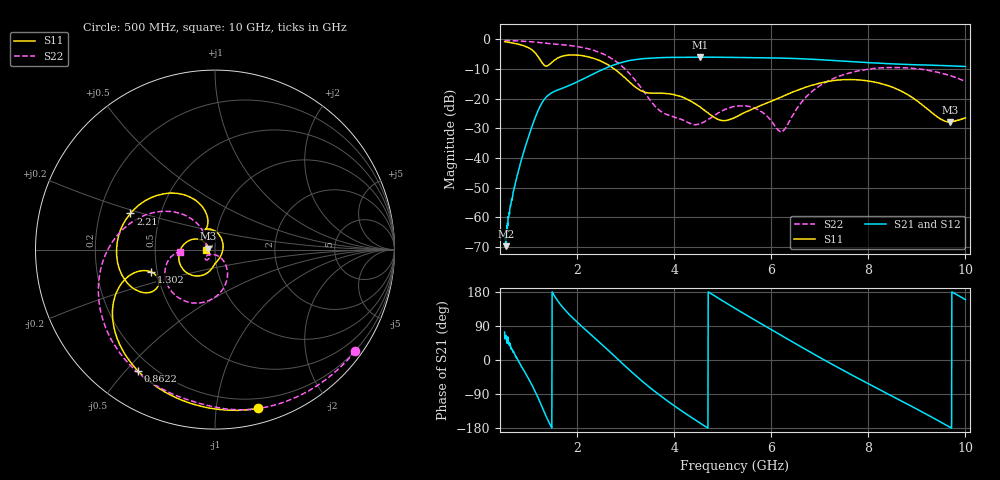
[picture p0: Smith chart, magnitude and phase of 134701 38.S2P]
!  2-Port S-parameters saved by WinCal
! VAR MeasName=S-Parameters (CALIBRATED_DATA) read from VNA (N5242A)
! VAR MeasDate=2013-7-3 16:37:20
! VAR NAME=134701 38
! VAR FILENAME=134701 38.S2P
! VAR DATE=2013-7-3 16:37:20
! VAR PHYS_PORTS=1,2
# Hz S MA R 50
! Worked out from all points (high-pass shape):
!   1601 points, 500 MHz to 10 GHz, reference 50 ohm
!   highest |S21| = -5.95 dB at 4.526 GHz (marker M1); lowest = -69.7 dB at 523.8 MHz (marker M2)
!   |S21| within 3 dB of the highest: 2.689 GHz to 9.74 GHz (7.051 GHz wide, 113 % of centre)
!   lowest |S11| = -27.8 dB at 9.679 GHz (marker M3), VSWR 1.08, Z = 46.1 + j0.538 ohm
!   |S11| at or under -10 dB: 2.768 GHz to end of sweep
!   |S22| runs from -31.1 to -0.3 dB; largest |S21 - S12| = 0.0022
!   S11 on the Smith chart (normalised r, x): 500 MHz: 0.12, -1.30; 862.2 MHz: 0.14, -0.54; 1.302 GHz: 0.46, -0.13; 2.21 GHz: 0.33, +0.18; 10 GHz: 0.91, -0.00
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5e8  0.9177 -74.7  0.0005114 73.8  0.0003456 81.2  0.9633 -35.9
5.2375e8  0.9114 -77.9  0.0003263 58.4  0.0005193 47.3  0.9615 -37.6
6.425e8  0.8793 -93.9  0.00202 27.8  0.001907 31.7  0.9547 -46.0
8.621875e8  0.8004 -122.5  0.01042 -19.9  0.0103 -20.5  0.9379 -61.6
1.075938e9  0.6564 -150.2  0.03632 -69.0  0.03631 -69.2  0.9131 -76.9
1.301562e9  0.3781 -160.9  0.09357 -132.9  0.09339 -133.0  0.8705 -92.4
1.598438e9  0.489 -152.0  0.1412 155.5  0.1408 155.2  0.8287 -111.9
2.085312e9  0.5356 167.2  0.2089 89.3  0.2079 89.1  0.7379 -147.7
2.21e9  0.5123 156.8  0.2346 75.0  0.2334 75.0  0.7011 -157.6
2.643438e9  0.3706 122.7  0.3448 24.8  0.3438 24.9  0.5131 165.7
2.981875e9  0.2252 104.6  0.4247 -15.6  0.4241 -15.5  0.3184 138.5
3.670625e9  0.1244 115.1  0.4933 -90.3  0.4922 -90.3  0.06606 140.2
4.525625e9  0.07319 61.7  0.504 -166.2  0.5034 -166.2  0.03746 -147.7
4.94125e9  0.0437 -0.5  0.5017 160.3  0.5017 160.4  0.05969 -124.5
5.25e9  0.04853 -51.6  0.4981 136.3  0.4983 136.3  0.07444 -129.0
5.719062e9  0.07334 -86.3  0.4922 101.0  0.4928 101.0  0.06574 -141.9
6.211875e9  0.1077 -99.9  0.4851 64.3  0.4856 64.3  0.02773 -98.2
6.835312e9  0.1688 -120.5  0.4646 18.4  0.4648 18.4  0.1325 -59.1
7.684375e9  0.2104 -159.6  0.421 -41.3  0.4209 -41.5  0.2826 -95.6
8.420625e9  0.1648 165.5  0.3913 -90.9  0.3894 -91.0  0.3363 -127.0
9.679375e9  0.04056 171.8  0.3593 -177.2  0.3583 -177.2  0.247 -170.9
1e10  0.04745 -178.7  0.3505 159.4  0.3497 159.5  0.1965 -176.8
